[IBIS ver]   5.0
[File name]  ddr_pba_ex.ibs
[File Rev]   1.0
[Date]   October 24, 2012
[Source]   Generic memory device
[Notes]   Created memory controller from a memory device
[Disclaimer]  Just an example file
[Copyright]   Copyright 2012 Cadence Design Systems, Inc. All rights reserved.
[Component]   Memory
[Manufacturer]  Cadence Design Systems, Inc.
[Package]
| variable   typ   min   max
R_pkg   1.0146   0.97286   1.0957
L_pkg   7.151e-9   6.591e-9   7.955e-9
C_pkg   3.058e-12   2.634e-12   3.335e-12
[Pin]   signal_name model_name   R_pin   L_pin   C_pin
A1   VDDQ   POWER
A2   DQ13   DQ   340.00m   1.53nH   0.52pF
A3   DQ15   DQ   260.00m   1.29nH   0.40pF
A7   DQ12   DQ   235.00m   1.19nH   0.38pF
A8   VDDQ   POWER
A9   VSS   GND
B1   VSSQ   GND
B2   VDD   POWER
B3   VSS   GND
B7   UDQS#   DQS   245.00m   1.18nH   0.38pF
B8   DQ14   DQ   317.00m   1.41nH   0.49pF
B9   VSSQ   GND
C1   VDDQ   POWER
C2   DQ11   DQ   301.00m   1.30nH   0.46pF
C3   DQ9   DQ   223.00m   1.07nH   0.36pF
C7   UDQS   DQS   225.00m   1.09nH   0.36pF
C8   DQ10   DQ   313.00m   1.31nH   0.47pF
C9   VDDQ   POWER
D1   VSSQ   GND
D2   VDDQ   POWER
D3   UDM   DM   218.00m   1.24nH   0.33pF
D7   DQ8   DQ   209.00m   0.96nH   0.34pF
D8   VSSQ   GND
D9   VDD   POWER
E1   VSS   GND
E2   VSSQ   GND
E3   DQ0   DQ   204.00m   1.02nH   0.33pF
E7   LDM   DM   195.00m   1.10nH   0.31pF
E8   VSSQ   GND
E9   VDDQ   POWER
F1   VDDQ   POWER
F2   DQ2   DQ   285.00m   1.30nH   0.43pF
F3   LDQS   DQS   234.00m   1.12nH   0.37pF
F7   DQ1   DQ   198.00m   0.96nH   0.32pF
F8   DQ3   DQ   284.00m   1.23nH   0.44pF
F9   VSSQ   GND
G1   VSSQ   GND
G2   DQ6   DQ   284.00m   1.23nH   0.43pF
G3   LDQS#   DQS   234.00m   1.11nH   0.37pF
G7   VDD   POWER
G8   VSS   GND
G9   VSSQ   GND
H1   VREFDQ   POWER
H2   VDDQ   POWER
H3   DQ4   DQ   194.00m   0.93nH   0.31pF
H7   DQ7   DQ   201.00m   1.00nH   0.33pF
H8   DQ5   DQ   271.00m   1.15nH   0.42pF
H9   VDDQ   POWER
J1   NC   NC
J2   VSS   GND
J3   RAS#   CTRL   198.00m   1.14nH   0.32pF
J7   CK   CLK   218.00m   1.15nH   0.34pF
J8   VSS   GND
J9   NC   NC
K1   ODT   CTRL   353.00m   1.14nH   0.52pF
K2   VDD   POWER
K3   CAS#   CTRL   205.00m   1.06nH   0.30pF
K7   CK#   CLK   215.00m   1.24nH   0.33pF
K8   VDD   POWER
K9   CKE   CTRL   369.00m   2.33nH   0.53pF
L1   NC   NC
L2   CS#   CTRL   274.00m   1.80nH   0.39pF
L3   WE#   CTRL   213.00m   1.33nH   0.31pF
L7   A10   CTRL   207.00m   1.24nH   0.31pF
L8   ZQ   NC   298.00m   1.62nH   0.46pF
L9   NC   NC
M1   VSS   GND
M2   BA0   CTRL   297.00m   1.48nH   0.43pF
M3   BA2   CTRL   200.00m   1.09nH   0.30pF
M7   NC   NC
M8   VREFCA   POWER
M9   VSS   GND
N1   VDD   POWER
N2   A3   CTRL   302.00m   1.86nH   0.45pF
N3   A0   CTRL   214.00m   1.14nH   0.33pF
N7   A12   CTRL   233.00m   1.33nH   0.36pF
N8   BA1   CTRL   326.00m   1.98nH   0.48pF
N9   VDD   POWER
P1   VSS   GND
P2   A5   CTRL   300.00m   1.94nH   0.44pF
P3   A2   CTRL   231.00m   1.53nH   0.34pF
P7   A1   CTRL   245.00m   1.65nH   0.37pF
P8   A4   CTRL   323.00m   2.07nH   0.48pF
P9   VSS   GND
R1   VDD   POWER
R2   A7   CTRL   338.00m   2.21nH   0.50pF
R3   A9   CTRL   271.00m   1.81nH   0.40pF
R7   A11   CTRL   268.00m   1.74nH   0.39pF
R8   A6   CTRL   346.00m   2.32nH   0.50pF
R9   VDD   POWER
T1   VSS   GND
T2   RST#   CTRL   421.00m   1.65nH   0.60pF
T3   A13   CTRL   322.00m   2.11nH   0.47pF
T7   NC   NC
T8   A8   CTRL   392.00m   2.58nH   0.57pF
T9   VSS   GND
|***********************PIN MAPPING*****************************************
[Pin Mapping] pulldown_ref pullup_ref gnd_clamp_ref power_clamp_ref ext_ref
A1   NC   PWRBUS2   |PWRBUS1 is VDD
A2   GNDBUS2   PWRBUS2   GNDBUS2   PWRBUS2 |PWRBUS2 is VDDQ
A3   GNDBUS2   PWRBUS2   GNDBUS2   PWRBUS2 |GNDBUS2 is VSSQ
A7   GNDBUS2   PWRBUS2   GNDBUS2   PWRBUS2
A8   NC   PWRBUS2
A9   GNDBUS1   NC
B1   GNDBUS2   NC
B2   NC   PWRBUS1   |GNDBUS1 is VSS
B3   GNDBUS1   NC
B7   GNDBUS2   PWRBUS2   GNDBUS2   PWRBUS2
B8   GNDBUS2   PWRBUS2   GNDBUS2   PWRBUS2
B9   GNDBUS2   NC
C1   NC   PWRBUS2
C2   GNDBUS2   PWRBUS2   GNDBUS2   PWRBUS2
C3   GNDBUS2   PWRBUS2   GNDBUS2   PWRBUS2
C7   GNDBUS2   PWRBUS2   GNDBUS2   PWRBUS2
C8   GNDBUS2   PWRBUS2   GNDBUS2   PWRBUS2
C9   NC   PWRBUS2
D1   GNDBUS2   NC
D2   NC   PWRBUS2
D3   GNDBUS2   PWRBUS2   GNDBUS2   PWRBUS2
D7   GNDBUS2   PWRBUS2   GNDBUS2   PWRBUS2
D8   GNDBUS2   NC
D9   NC   PWRBUS1
E1   GNDBUS1   NC
E2   GNDBUS2   NC
E3   GNDBUS2   PWRBUS2   GNDBUS2   PWRBUS2
E7   GNDBUS2   PWRBUS2   GNDBUS2   PWRBUS2
E8   GNDBUS2   NC
E9   NC   PWRBUS2
F1   NC   PWRBUS2
F2   GNDBUS2   PWRBUS2   GNDBUS2   PWRBUS2
F3   GNDBUS2   PWRBUS2   GNDBUS2   PWRBUS2
F7   GNDBUS2   PWRBUS2   GNDBUS2   PWRBUS2
F8   GNDBUS2   PWRBUS2   GNDBUS2   PWRBUS2
F9   GNDBUS2   NC
G1   GNDBUS2   NC
G2   GNDBUS2   PWRBUS2   GNDBUS2   PWRBUS2
G3   GNDBUS2   PWRBUS2   GNDBUS2   PWRBUS2
G7   NC   PWRBUS1
G8   GNDBUS1   NC
G9   GNDBUS2   NC
H1   NC   REFDQ   |VREFDQ
H2   NC   PWRBUS2
H3   GNDBUS2   PWRBUS2   GNDBUS2   PWRBUS2
H7   GNDBUS2   PWRBUS2   GNDBUS2   PWRBUS2
H8   GNDBUS2   PWRBUS2   GNDBUS2   PWRBUS2
H9   NC   PWRBUS2
J1   NC   NC
J2   GNDBUS1   NC
J3   GNDBUS1   PWRBUS1   GNDBUS1   PWRBUS1
J7   GNDBUS1   PWRBUS1   GNDBUS1   PWRBUS1
J8   GNDBUS1   NC
J9   NC   NC
K1   GNDBUS1   PWRBUS1   GNDBUS1   PWRBUS1
K2   NC   PWRBUS1
K3   GNDBUS1   PWRBUS1   GNDBUS1   PWRBUS1
K7   GNDBUS1   PWRBUS1   GNDBUS1   PWRBUS1
K8   NC   PWRBUS1
K9   GNDBUS1   PWRBUS1   GNDBUS1   PWRBUS1
L1   NC   NC
L2   GNDBUS1   PWRBUS1   GNDBUS1   PWRBUS1
L3   GNDBUS1   PWRBUS1   GNDBUS1   PWRBUS1
L7   GNDBUS1   PWRBUS1   GNDBUS1   PWRBUS1
L8   NC   NC
L9   NC   NC
M1   GNDBUS1   NC
M2   GNDBUS1   PWRBUS1   GNDBUS1   PWRBUS1
M3   GNDBUS1   PWRBUS1   GNDBUS1   PWRBUS1
M7   NC   NC
M8   NC   REFCA   |VREFCA
M9   GNDBUS1   NC
N1   NC   PWRBUS1
N2   GNDBUS1   PWRBUS1   GNDBUS1   PWRBUS1
N3   GNDBUS1   PWRBUS1   GNDBUS1   PWRBUS1
N7   GNDBUS1   PWRBUS1   GNDBUS1   PWRBUS1
N8   GNDBUS1   PWRBUS1   GNDBUS1   PWRBUS1
N9   NC   PWRBUS1
P1   GNDBUS1   NC
P2   GNDBUS1   PWRBUS1   GNDBUS1   PWRBUS1
P3   GNDBUS1   PWRBUS1   GNDBUS1   PWRBUS1
P7   GNDBUS1   PWRBUS1   GNDBUS1   PWRBUS1
P8   GNDBUS1   PWRBUS1   GNDBUS1   PWRBUS1
P9   GNDBUS1   NC
R1   NC   PWRBUS1
R2   GNDBUS1   PWRBUS1   GNDBUS1   PWRBUS1
R3   GNDBUS1   PWRBUS1   GNDBUS1   PWRBUS1
R7   GNDBUS1   PWRBUS1   GNDBUS1   PWRBUS1
R8   GNDBUS1   PWRBUS1   GNDBUS1   PWRBUS1
R9   NC   PWRBUS1
T1   GNDBUS1   NC
T2   GNDBUS1   PWRBUS1   GNDBUS1   PWRBUS1
T3   GNDBUS1   PWRBUS1   GNDBUS1   PWRBUS1
T7   NC   NC
T8   GNDBUS1   PWRBUS1   GNDBUS1   PWRBUS1
T9   GNDBUS1   NC
|**********************DIFF PIN*********************************************
[Diff_pin]   inv_pin   vdiff   tdelay_typ   tdelay_min   tdelay_max
   F3   G3   0.350V   0ns   NA   NA
   C7   B7   0.350V   0ns   NA   NA
   J7   K7   0.350V   0ns   NA   NA
|**********************Component Bus Definitions ***************************
|[Component Type]   Memory
|[Bus Type]   AddCmd
|TimingRef   CK / CK#
|EdgeType   RiseEdge
|MinReceiveSetup   0.2UI
|MinReceiveHold   0.2UI
|SignalName   A0 A1 A2 A3 A4 A5 A6 A7
|[Bus Type]   Data
|BusGroup   DataL
|TimingRef   LDQS / LDQS#
|EdgeType   BothEdges
|MinReceiveSetup   0.1UI
|MinReceiveHold   0.1UI
|tDQSQ   0.1UI
|tQH   0.9UI
|SignalName   DQ0 DQ1 DQ2 DQ3 DQ4 DQ5 DQ6 DQ7
|[Bus Type]   Data
|BusGroup   DataU
|TimingRef   UDQS / UDQS#
|EdgeType   BothEdges
|MinReceiveSetup   0.1UI
|MinReceiveHold   0.1UI
|tDQSQ   0.1UI
|tQH   0.9UI
|SignalName   DQ8 DQ9 DQ10 DQ11 DQ12 DQ13 DQ14 DQ15
[Component]   Controller
[Manufacturer]  Cadence Design Systems, Inc.
[Package]
| variable   typ   min   max
R_pkg   1.0146   0.97286   1.0957
L_pkg   7.151e-9   6.591e-9   7.955e-9
C_pkg   3.058e-12   2.634e-12   3.335e-12
[Pin]  signal_name   model_name   R_pin   L_pin   C_pin
1   VDD   POWER
2   CLK1N   CLK
3   CLK1P   CLK
4   DNU   NC
5   VSS   GND
6   VDD   POWER
7   DNU   NC
8   VSS   GND
9   VDD   POWER
10   RESET   CTRL
11   DNU   NC
12   A13   ADDR
13   A11   ADDR
14   A9   ADDR
15   A7   ADDR
16   A8   ADDR
17   A2   ADDR
18   A6   ADDR
19   A5   ADDR
20   A1   ADDR
21   A3   ADDR
22   A4   ADDR
23   A0   ADDR
24   VSS   GND
25   VDD   POWER
26   BA1   ADDR
27   A12   ADDR
28   BA0   ADDR
29   BA2   ADDR
30   VDD   POWER
31   VSS   GND
32   CLK2N   CLK
33   CLK2P   CLK
34   VREFCA   POWER
35   DNU   NC
36   VDDQ   POWER
37   ZQ   CTRL
38   VSSQ   GND
39   A10   ADDR
40   VSS   GND
41   VDD   POWER
42   CLK3N   CLK
43   CLK3P   CLK
44   DNU   NC
45   WE   CTRL
46   CS   CTRL
47   ODT   CTRL
48   DNU   NC
49   CKE   CTRL
50   DNU   NC
51   CLK0N   CLK
52   CLK0P   CLK
53   VDD   POWER
54   VSS   GND
55   CAS   CTRL
56   VDDDLL   POWER
57   VSSDL   GND
58   RAS   CTRL
59   DNU   NC
60   VREFDQ   POWER
61   VSSQ   GND
62   DQ4   DQ
63   VDDQ   POWER
64   DQ6   DQ
65   VSSQ   GND
66   VSSQ   GND
67   DQ7   DQ
68   VDDQ   POWER
69   DQ5   DQ
70   VSS   GND
71   VSSQ   GND
72   VDD   POWER
73   VSS   GND
74   VSSQ   GND
75   LDQS#   DQS
76   VDDQ   POWER
77   LDQS   DQS
78   VSSQ   GND
79   VSSQ   GND
80   DQ1   DQ
81   VDDQ   POWER
82   DQ3   DQ
83   VSSQ   GND
84   VSSQ   GND
85   DQ2   DQ
86   VDDQ   POWER
87   DQ0   DQ
88   VSSQ   GND
89   LDM   DQ
90   VDD   POWER
91   VSS   GND
92   UDM   DQ
93   VDDQ   POWER
94   DQ8   DQ
95   VSSQ   GND
96   DQ10   DQ
97   VDDQ   POWER
98   VDDQ   POWER
99   DQ11   DQ
100   VSSQ   GND
101   DQ9   DQ
102   VDDQ   POWER
103   VDDQ   POWER
104   UDQS   DQS
105   VSSQ   GND
106   UDQS#   DQS
107   VDDQ   POWER
108   VDD   POWER
109   VSS   GND
110   VDDQ   POWER
111   DQ13   DQ
112   VSSQ   GND
113   DQ15   DQ
114   VDDQ   POWER
115   VDDQ   POWER
116   DQ14   DQ
117   VSSQ   GND
118   DQ12   DQ
119   VDDQ   POWER
120   DNU   NC
[Pin Mapping]   pulldown_ref   pullup_ref  gnd_clamp_ref   power_clamp_ref ext_ref
1   NC   PWRBUS1
2   GNDBUS1   PWRBUS1   GNDBUS1   PWRBUS1
3   GNDBUS1   PWRBUS1   GNDBUS1   PWRBUS1
4   NC   NC
5   GNDBUS1   NC
6   NC   PWRBUS1
7   NC   NC
8   GNDBUS1   NC
9   NC   PWRBUS1
10   GNDBUS1   PWRBUS1   GNDBUS1   PWRBUS1
11   NC   NC
12   GNDBUS1   PWRBUS1   GNDBUS1   PWRBUS1
13   GNDBUS1   PWRBUS1   GNDBUS1   PWRBUS1
14   GNDBUS1   PWRBUS1   GNDBUS1   PWRBUS1
15   GNDBUS1   PWRBUS1   GNDBUS1   PWRBUS1
16   GNDBUS1   PWRBUS1   GNDBUS1   PWRBUS1
17   GNDBUS1   PWRBUS1   GNDBUS1   PWRBUS1
18   GNDBUS1   PWRBUS1   GNDBUS1   PWRBUS1
19   GNDBUS1   PWRBUS1   GNDBUS1   PWRBUS1
20   GNDBUS1   PWRBUS1   GNDBUS1   PWRBUS1
21   GNDBUS1   PWRBUS1   GNDBUS1   PWRBUS1
22   GNDBUS1   PWRBUS1   GNDBUS1   PWRBUS1
23   GNDBUS1   PWRBUS1   GNDBUS1   PWRBUS1
24   GNDBUS1   NC
25   NC   PWRBUS1
26   GNDBUS1   PWRBUS1   GNDBUS1   PWRBUS1
27   GNDBUS1   PWRBUS1   GNDBUS1   PWRBUS1
28   GNDBUS1   PWRBUS1   GNDBUS1   PWRBUS1
29   GNDBUS1   PWRBUS1   GNDBUS1   PWRBUS1
30   NC   PWRBUS1
31   GNDBUS1   NC
32   GNDBUS1   PWRBUS1   GNDBUS1   PWRBUS1
33   GNDBUS1   PWRBUS1   GNDBUS1   PWRBUS1
34   NC   REFCA
35   NC   NC
36   NC   PWRBUS2
37   NC   NC
38   GNDBUS2   NC
39   GNDBUS1   PWRBUS1   GNDBUS1   PWRBUS1
40   GNDBUS1   NC
41   NC   PWRBUS1
42   GNDBUS1   PWRBUS1   GNDBUS1   PWRBUS1
43   GNDBUS1   PWRBUS1   GNDBUS1   PWRBUS1
44   NC   NC
45   GNDBUS1   PWRBUS1   GNDBUS1   PWRBUS1
46   GNDBUS1   PWRBUS1   GNDBUS1   PWRBUS1
47   GNDBUS1   PWRBUS1   GNDBUS1   PWRBUS1
48   NC   NC
49   GNDBUS1   PWRBUS1   GNDBUS1   PWRBUS1
50   NC   NC
51   GNDBUS1   PWRBUS1   GNDBUS1   PWRBUS1
52   GNDBUS1   PWRBUS1   GNDBUS1   PWRBUS1
53   NC   PWRBUS1
54   GNDBUS1   NC
55   GNDBUS1   PWRBUS1   GNDBUS1   PWRBUS1
56   NC   PWRBUS1
57   GNDBUS1   NC
58   GNDBUS1   PWRBUS1   GNDBUS1   PWRBUS1
59   NC   NC
60   NC   REFDQ
61   GNDBUS2   NC
62   GNDBUS2   PWRBUS2   GNDBUS2   PWRBUS2
63   NC   PWRBUS2
64   GNDBUS2   PWRBUS2   GNDBUS2   PWRBUS2
65   GNDBUS2   NC
66   GNDBUS2   NC
67   GNDBUS2   PWRBUS2   GNDBUS2   PWRBUS2
68   NC   PWRBUS2
69   GNDBUS2   PWRBUS2   GNDBUS2   PWRBUS2
70   GNDBUS1   NC
71   GNDBUS2   NC
72   NC   PWRBUS1
73   GNDBUS1   NC
74   GNDBUS2   NC
75   GNDBUS2   PWRBUS2   GNDBUS2   PWRBUS2
76   NC   PWRBUS2
77   GNDBUS2   PWRBUS2   GNDBUS2   PWRBUS2
78   GNDBUS2   NC
79   GNDBUS2   NC
80   GNDBUS2   PWRBUS2   GNDBUS2   PWRBUS2
81   NC   PWRBUS2
82   GNDBUS2   PWRBUS2   GNDBUS2   PWRBUS2
83   GNDBUS2   NC
84   GNDBUS2   NC
85   GNDBUS2   PWRBUS2   GNDBUS2   PWRBUS2
86   NC   PWRBUS2
87   GNDBUS2   PWRBUS2   GNDBUS2   PWRBUS2
88   GNDBUS2   NC
89   GNDBUS2   PWRBUS2   GNDBUS2   PWRBUS2
90   NC   PWRBUS1
91   GNDBUS1   NC
92   GNDBUS2   PWRBUS2   GNDBUS2   PWRBUS2
93   NC   PWRBUS2
94   GNDBUS2   PWRBUS2   GNDBUS2   PWRBUS2
95   GNDBUS2   NC
96   GNDBUS2   PWRBUS2   GNDBUS2   PWRBUS2
97   NC   PWRBUS2
98   NC   PWRBUS2
99   GNDBUS2   PWRBUS2   GNDBUS2   PWRBUS2
100   GNDBUS2   NC
101   GNDBUS2   PWRBUS2   GNDBUS2   PWRBUS2
102   NC   PWRBUS2
103   NC   PWRBUS2
104   GNDBUS2   PWRBUS2   GNDBUS2   PWRBUS2
105   GNDBUS2   NC
106   GNDBUS2   PWRBUS2   GNDBUS2   PWRBUS2
107   NC   PWRBUS2
108   NC   PWRBUS1
109   GNDBUS1   NC
110   NC   PWRBUS2
111   GNDBUS2   PWRBUS2   GNDBUS2   PWRBUS2
112   GNDBUS2   NC
113   GNDBUS2   PWRBUS2   GNDBUS2   PWRBUS2
114   NC   PWRBUS2
115   NC   PWRBUS2
116   GNDBUS2   PWRBUS2   GNDBUS2   PWRBUS2
117   GNDBUS2   NC
118   GNDBUS2   PWRBUS2   GNDBUS2   PWRBUS2
119   NC   PWRBUS2
120   NC   NC
[Diff_pin]   inv_pin   vdiff   tdelay_typ   tdelay_min   tdelay_max
   3   2   NA   0ns   NA   NA
   33   32   NA   0ns   NA   NA
   43   42   NA   0ns   NA   NA
   52   51   NA   0ns   NA   NA
   77   75   0.350V   0ns   NA   NA
   104   106   0.350V   0ns   NA   NA
|**********************Component Bus Definitions ***************************
|[Component Type]   Controller
|[Bus Type]   AddCmd
|BusGroup   Address
|TimingRef   CLK0P / CLK0N, CLK1P / CLK1N, CLK2P / CLK2N, CLK3P / CLK3N
|EdgeType   RiseEdge
|MinTransmitSetup   0.3125UI
|MinTransmitHold   0.3125UI
|SignalName   A0 A1 A2 A3 A4 A5 A6 A7
|[Bus Type]   Data
|BusGroup   DataL
|TimingRef   LDQS / LDQS#
|EdgeType   BothEdges
|SignalName   DQ0 DQ1 DQ2 DQ3 DQ4 DQ5 DQ6 DQ7
|[Bus Type]   Data
|BusGroup   DataU
|TimingRef   UDQS / UDQS#
|EdgeType   BothEdges
|SignalName   DQ8 DQ9 DQ10 DQ11 DQ12 DQ13 DQ14 DQ15
[Model Selector] DQ
DDR3_DQ34_NO_ODT   34Ohm DDR3  I/O DRIVER NO ODT
DDR3_DQ34_ODT   34Ohm DDR3  I/O DRIVER 60Ohm ODT
DDR3_DQ40_NO_ODT   40Ohm DDR3  I/O DRIVER NO ODT
DDR3_DQ40_ODT   40Ohm DDR3  I/O DRIVER 60Ohm ODT
DDR3_DQ48_NO_ODT   48Ohm DDR3  I/O DRIVER NO ODT
DDR3_DQ48_ODT   48Ohm DDR3  I/O DRIVER 60Ohm ODT
LPDDR2_DQ60   60Ohm LPDDR2 DRIVER
DDR3L_DQ40_NO_ODT   40Ohm DDR3L I/O DRIVER NO ODT
DDR3L_DQ40_ODT   40Ohm DDR3L I/O DRIVER 60Ohm ODT
DDR3L_DQ48_NO_ODT   48Ohm DDR3L I/O DRIVER NO ODT
DDR3L_DQ48_ODT   48Ohm DDR3L I/O DRIVER 60Ohm ODT
DDR4_DQ34N48P_NO_ODT   34N 48P DDR4 I/O DRIVER NO ODT
DDR4_DQ34N48P_ODT   34N 48P DDR4 I/O DRIVER 60Ohm ODT
DDR4_DQ34N60P_NO_ODT   34N 60P DDR4 I/O DRIVER NO ODT
DDR4_DQ34N60P_ODT   34N 48P DDR4 I/O DRIVER 60Ohm ODT
DDR4_DQ40N48P_NO_ODT   40N 48P DDR4 I/O DRIVER NO ODT
DDR4_DQ40N48P_ODT   40N 48P DDR4 I/O DRIVER 60Ohm ODT
DDR4_DQ40N60P_NO_ODT   40N 60P DDR4 I/O DRIVER NO ODT
DDR4_DQ40N60P_ODT   40N 60P DDR4 I/O DRIVER 60Ohm ODT
[Model Selector] DM
DDR3_DQ34_NO_ODT   34Ohm DDR3  I/O DRIVER NO ODT
DDR3_DQ40_NO_ODT   40Ohm DDR3  I/O DRIVER NO ODT
DDR3_DQ48_NO_ODT   48Ohm DDR3  I/O DRIVER NO ODT
LPDDR2_DQ60   60Ohm LPDDR2 DRIVER
DDR3L_DQ40_NO_ODT   40Ohm DDR3L I/O DRIVER NO ODT
DDR3L_DQ48_NO_ODT   48Ohm DDR3L I/O DRIVER NO ODT
DDR4_DQ34N48P_NO_ODT   34N 48P DDR4 I/O DRIVER NO ODT
DDR4_DQ34N60P_NO_ODT   34N 60P DDR4 I/O DRIVER NO ODT
DDR4_DQ40N48P_NO_ODT   40N 48P DDR4 I/O DRIVER NO ODT
DDR4_DQ40N60P_NO_ODT   40N 60P DDR4 I/O DRIVER NO ODT
[Model Selector] DQS
DDR3_DQS34_NO_ODT   34Ohm DDR3 I/O STROBE NO ODT
DDR3_DQS34_ODT   34Ohm DDR3 I/O STROBE 60Ohm ODT
DDR3_DQS40_NO_ODT   40Ohm DDR3  I/O STROBE NO ODT
DDR3_DQS40_ODT   40Ohm DDR3  I/O STROBE 60Ohm ODT
DDR3_DQS48_NO_ODT   48Ohm DDR3  I/O STROBE NO ODT
DDR3_DQS48_ODT   48Ohm DDR3  I/O STROBE 60Ohm ODT
LPDDR2_DQS60   60Ohm LPDDR2 STROBE
DDR3L_DQS40_NO_ODT   40Ohm DDR3L I/O STROBE NO ODT
DDR3L_DQS40_ODT   40Ohm DDR3L I/O STROBE 60Ohm ODT
DDR3L_DQS48_NO_ODT   48Ohm DDR3L I/O STROBE NO ODT
DDR3L_DQS48_ODT   48Ohm DDR3L I/O STROBE 60Ohm ODT
DDR4_DQS34N48P_NO_ODT  34N 48P DDR4 I/O STROBE NO ODT
DDR4_DQS34N48P_ODT   34N 48P DDR4 I/O STROBE 60Ohm ODT
DDR4_DQS34N60P_NO_ODT  34N 60P DDR4 I/O STROBE NO ODT
DDR4_DQS34N60P_ODT   34N 48P DDR4 I/O STROBE 60Ohm ODT
DDR4_DQS40N48P_NO_ODT  40N 48P DDR4 I/O STROBE NO ODT
DDR4_DQS40N48P_ODT   40N 48P DDR4 I/O STROBE 60Ohm ODT
DDR4_DQS40N60P_NO_ODT  40N 60P DDR4 I/O STROBE NO ODT
DDR4_DQS40N60P_ODT   40N 60P DDR4 I/O STROBE 60Ohm ODT
[Model Selector] ADDR
DDR3_DQ34_NO_ODT   34Ohm DDR3  I/O DRIVER
DDR3_DQ40_NO_ODT   40Ohm DDR3  I/O DRIVER
DDR3_DQ48_NO_ODT   48Ohm DDR3  I/O DRIVER
LPDDR2_DQ60   60Ohm LPDDR2 DRIVER
DDR3L_DQ40_NO_ODT   40Ohm DDR3L I/O DRIVER
DDR3L_DQ48_NO_ODT   48Ohm DDR3L I/O DRIVER
DDR4_DQ34N48P_NO_ODT   34N 48P DDR4 I/O DRIVER
DDR4_DQ34N60P_NO_ODT   34N 60P DDR4 I/O DRIVER
DDR4_DQ40N48P_NO_ODT   40N 48P DDR4 I/O DRIVER
DDR4_DQ40N60P_NO_ODT   40N 60P DDR4 I/O DRIVER
[Model Selector] CTRL
DDR3_DQ34_NO_ODT   34Ohm DDR3  I/O DRIVER
DDR3_DQ40_NO_ODT   40Ohm DDR3  I/O DRIVER
DDR3_DQ48_NO_ODT   48Ohm DDR3  I/O DRIVER
LPDDR2_DQ60   60Ohm LPDDR2 DRIVER
DDR3L_DQ40_NO_ODT   40Ohm DDR3L I/O DRIVER
DDR3L_DQ48_NO_ODT   48Ohm DDR3L I/O DRIVER
DDR4_DQ34N48P_NO_ODT   34N 48P DDR4 I/O DRIVER
DDR4_DQ34N60P_NO_ODT   34N 60P DDR4 I/O DRIVER
DDR4_DQ40N48P_NO_ODT   40N 48P DDR4 I/O DRIVER
DDR4_DQ40N60P_NO_ODT   40N 60P DDR4 I/O DRIVER
[Model Selector] CLK
DDR3_DQS34_NO_ODT   34Ohm DDR3 I/O CLOCK
DDR3_DQS40_NO_ODT   40Ohm DDR3  I/O CLOCK
DDR3_DQS48_NO_ODT   48Ohm DDR3  I/O CLOCK
LPDDR2_DQS60   60Ohm LPDDR2 CLOCK
DDR3L_DQS40_NO_ODT   40Ohm DDR3L I/O CLOCK
DDR3L_DQS48_NO_ODT   48Ohm DDR3L I/O CLOCK
DDR4_DQS34N48P_NO_ODT  34N 48P DDR4 I/O CLOCK
DDR4_DQS34N60P_NO_ODT  34N 60P DDR4 I/O CLOCK
DDR4_DQS40N48P_NO_ODT  40N 48P DDR4 I/O CLOCK
DDR4_DQS40N60P_NO_ODT  40N 60P DDR4 I/O CLOCK
| Models and submodels in the file (44): DDR3L_DQ40_NO_ODT (I/O), DDR3L_DQ40_ODT (I/O), DDR3L_DQ48_NO_ODT (I/O), DDR3L_DQ48_ODT (I/O), DDR3L_DQS40_NO_ODT (I/O), DDR3L_DQS40_ODT (I/O), DDR3L_DQS48_NO_ODT (I/O), DDR3L_DQS48_ODT (I/O), DDR3_DQ34_NO_ODT (I/O), DDR3_DQ34_ODT (I/O), DDR3_DQ40_NO_ODT (I/O), DDR3_DQ40_ODT (I/O), DDR3_DQ48_NO_ODT (I/O), DDR3_DQ48_ODT (I/O), DDR3_DQS34_NO_ODT (I/O), DDR3_DQS34_ODT (I/O), DDR3_DQS40_NO_ODT (I/O), DDR3_DQS40_ODT (I/O), DDR3_DQS48_NO_ODT (I/O), DDR3_DQS48_ODT (I/O), DDR4_DQ34N48P_NO_ODT (I/O), DDR4_DQ34N48P_ODT (I/O), DDR4_DQ34N60P_NO_ODT (I/O), DDR4_DQ34N60P_ODT (I/O), DDR4_DQ40N48P_NO_ODT (I/O), DDR4_DQ40N48P_ODT (I/O), DDR4_DQ40N60P_NO_ODT (I/O), DDR4_DQ40N60P_ODT (I/O), DDR4_DQS34N48P_NO_ODT (I/O), DDR4_DQS34N48P_ODT (I/O), DDR4_DQS34N60P_NO_ODT (I/O), DDR4_DQS34N60P_ODT (I/O), DDR4_DQS40N48P_NO_ODT (I/O), DDR4_DQS40N48P_ODT (I/O), DDR4_DQS40N60P_NO_ODT (I/O), DDR4_DQS40N60P_ODT (I/O), LPDDR2_DQ60 (I/O), LPDDR2_DQS60 (I/O), DDR3_DQ_ODT60 (Dynamic_clamp), DDR3_DQS_ODT60 (Dynamic_clamp), DDR3L_DQ_ODT60 (Dynamic_clamp), DDR3L_DQS_ODT60 (Dynamic_clamp), DDR4_DQ_ODT60 (Dynamic_clamp), DDR4_DQS_ODT60 (Dynamic_clamp)
